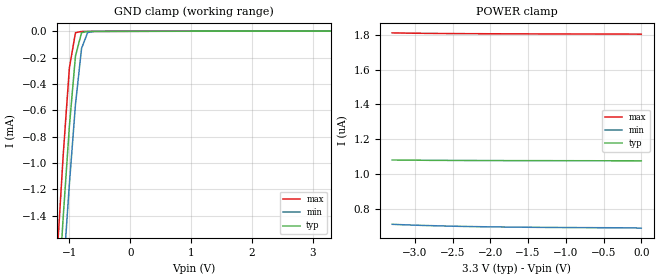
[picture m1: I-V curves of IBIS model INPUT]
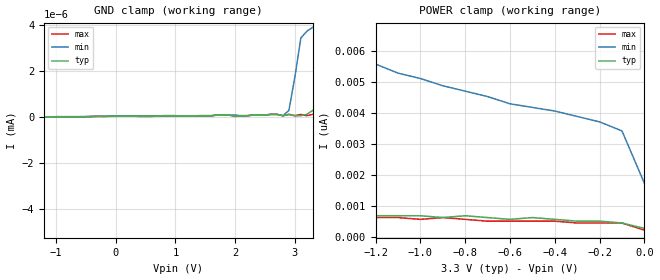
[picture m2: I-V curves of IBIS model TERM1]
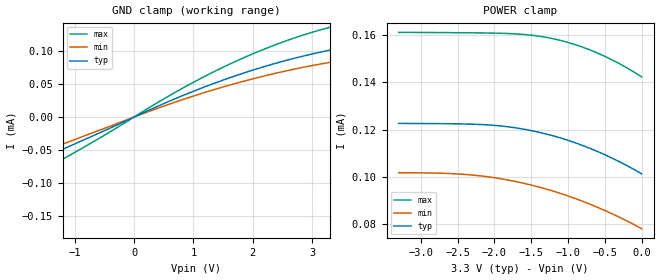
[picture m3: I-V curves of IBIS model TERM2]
|   PERICOM SEMICONDUCTOR CORP
|   IBIS Model of PI3USB223
|   Product Family: 3USB
|   UQFN (ZM) Package
[IBIS Ver] 3.2
[Comment char] |_char
[File Name] pi3usb223_zm_33v.ibs
[File Rev] 1.0
[Source] File originated at Pericom Semiconductor Corp.
[Date] 9/17/15
[Disclaimer] (C) Copyright PERICOM Semiconductor Corporation
   All rights reserved
  Pericom Semiconductor Corporation hereby grants the user of
  this IBIS model a non-exclusive, nontransferable license to
  use this IBIS model under the following terms.
  This IBIS model is provided on an "AS IS" basis and Pericom
  makes absolutely no warranty with respect to the information
  contained herein. PERICOM DISCLAIMS AND CUSTOMER WAIVES ALL
  WARRANTIES, EXPRESSED OR IMPLIED, INCLUDING WARRANTIES OF
  MERCHANTABILITY OR FITNESS FOR A PARTICULAR PURPOSE. The
  entire risk as to quality and performance is with the customer.
  Accordingly, in no event shall the company be liable for any
  damages, whether in contract or tort, including any lost
  profits or other incidental, consequential, exemplary, or
  punitive damages arising out of the use or application of the
  IBIS model provided in this package. Further, Pericom reserves
  the right to make changes without notice to any product herein
  to improve reliability, function, or design. Pericom does not
  convey any license under patent rights or any other intellectual
  property rights, including those of third parties.
  The user is granted this license only to use the IBIS model
  and is not granted rights to sell, load, rent, lease or license
  the IBIS model in whole or in part, or in modified form to anyone
  other than user. User may modify the IBIS model to suit its specific
  application but rights to derivative works and such modifications
  shall belong to Pericom.
  Pericom is not obligated to provide maintenance or support
  for the licensed IBIS model.
  Contact Pericom at ATTN: APPLICATION ENGINEERING / IBIS MODELS
  1545 Barber Lane Milpitas, CA 95035 USA.
[Component] PI3USB223
[Manufacturer] Pericom Semiconductor Corp.
[Package]
| variable   typ   min   max
R_pkg   0.028337ohm   0.027528ohm   0.029145ohm
L_pkg   0.39561nH   0.38133nH   0.40988nH
C_pkg   0.047513pF   0.038136pF   0.056889pF
[Pin]   signal_name   model_name   R_pin   L_pin   C_pin
1   D-   TERM1   0.027896   0.38515nH   0.041595pF
2   R   TERM2   0.027896   0.38515nH   0.041595pF
3   L   TERM2   0.029145   0.40988nH   0.056889pF
4   GND   GND   0.027528   0.38133nH   0.038136pF
5   VDD   POWER   0.029145   0.40988nH   0.056889pF
6   D-/L   TERM3   0.027896   0.38515nH   0.041595pF
7   D+/R   TERM3   0.027896   0.38515nH   0.041595pF
8   ASEL   INPUT   0.029145   0.40988nH   0.056889pF
9   VBUS   INPUT   0.027528   0.38133nH   0.038136pF
10   D+   TERM1   0.029145   0.40988nH   0.056889pF
[Series Switch Groups]
On 1 /
Off 2 /
[Series Pin Mapping]   pin_2   model_name  function_table_group
1   6   SWITCH1   1
10   7   SWITCH1   1
2   6   SWITCH2   2
3   7   SWITCH2   2
|   Model SWITCH1
[Model] SWITCH1
Model_type Series_switch
| variable   typ   min   max
C_comp   7.000pF   6.900pF   7.100pF
[Voltage Range]   3.300V   3.000V   3.600V
[GND Clamp Reference]   0.000V   0.000V   0.000V
[POWER Clamp Reference]   3.300V   3.000V   3.600V
[On]
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[OFF]
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|   Model SWITCH2
[Model] SWITCH2
Model_type Series_switch
| variable   typ   min   max
C_comp   7.000pF   6.900pF   7.100pF
[Voltage Range]   3.300V   3.000V   3.600V
[GND Clamp Reference]   0.000V   0.000V   0.000V
[POWER Clamp Reference]   3.300V   3.000V   3.600V
[On]
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[OFF]
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| Models and submodels in the file (6): INPUT (Input), SWITCH1 (Series_switch), SWITCH2 (Series_switch), TERM1 (Terminator), TERM2 (Terminator), TERM3 (Terminator)
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|   Model INPUT
[Model] INPUT
Model_type Input
Vinl = 0.800V
Vinh = 2.000V
| variable   typ   min   max
C_comp   1.000pF   0.900pF   1.100pF
[Voltage Range]   3.300V   3.000V   3.600V
[GND Clamp Reference]   0.000V   0.000V   0.000V
[POWER Clamp Reference]   3.300V   3.000V   3.600V
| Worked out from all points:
|   GND clamp passes 1 mA (typ) near -1.04 V on its own axis
[GND Clamp]
| Voltage   I(typ)   I(min)   I(max)
-3.3V     -19.61mA   -19.28mA   -20.05mA
-1.2V     -2.136mA   -2.542mA   -1.694mA
-1.1V     -1.403mA   -1.835mA   -931.7uA
-1V       -721.6uA   -1.161mA   -278uA
-900mV    -187.7uA   -555.9uA   -10.55uA
-800mV    -10.15uA   -129.5uA   -1.14uA
-700mV    -880.6nA   -9.377uA   -929.6nA
-500mV    -459.5nA   -365.8nA   -657.3nA
3.3V      1.076uA    692.4nA    1.803uA
[POWER Clamp]   |Note: Vtable = Vcc - Voutput
| Voltage   I(typ)   I(min)   I(max)
-3.3V     1.081uA    712.6nA    1.81uA
-3.2V     1.081uA    710.6nA    1.81uA
-3.1V     1.08uA     709.1nA    1.809uA
-3V       1.08uA     707.6nA    1.808uA
-2.8V     1.079uA    704.9nA    1.808uA
-2.5V     1.079uA    701.6nA    1.806uA
-2.1V     1.078uA    698.4nA    1.805uA
-1.5V     1.077uA    695.5nA    1.805uA
-1.3V     1.077uA    694.8nA    1.804uA
-1V       1.077uA    693.9nA    1.804uA
-100mV    1.077uA    691.9nA    1.803uA
0V        1.076uA    690.3nA    1.803uA
|   Model TERM1
[Model] TERM1
Model_type Terminator
| variable   typ   min   max
C_comp   3.000pF   2.950pF   3.050pF
[Voltage Range]   3.300V   3.000V   3.600V
[GND Clamp Reference]   0.000V   0.000V   0.000V
[POWER Clamp Reference]   3.300V   3.000V   3.600V
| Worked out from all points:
|   GND clamp passes 1 mA (typ) near -2.90 V on its own axis
[GND Clamp]
| Voltage   I(typ)   I(min)   I(max)
-3.3V     -1.584A    -1.988A    -1.092A
-2.5V     -307nA     -2.561uA   -8.702nA
-2.4V     -10.74nA   -165.2nA   -116.4pA
-2.3V     -349.2pA   -8.702nA   0A
-2.2V     -58.21pA   -407.5pA   0A
-2.1V     0A         -58.21pA   0A
2.6V      116.4pA    116.4pA    116.4pA
2.8V      58.21pA    58.21pA    58.21pA
2.9V      116.4pA    291pA      116.4pA
3V        58.21pA    1.746nA    58.21pA
3.1V      58.21pA    3.434nA    116.4pA
3.3V      291pA      3.9nA      116.4pA
[POWER Clamp]   |Note: Vtable = Vcc - Voutput
| Voltage   I(typ)   I(min)   I(max)
-3.3V     1.63nA     21.77nA    1.048nA
-3.1V     1.513nA    18.86nA    814.9pA
-2.9V     1.513nA    16.18nA    814.9pA
-2.8V     1.281nA    15.02nA    931.3pA
-2.6V     1.164nA    13.04nA    931.3pA
-2.5V     1.164nA    11.99nA    698.5pA
-2.2V     931.3pA    9.895nA    814.9pA
-2.1V     1.048nA    9.313nA    698.5pA
-1.5V     873.1pA    6.519nA    640.3pA
-1.1V     698.5pA    5.297nA    640.3pA
-100mV    465.7pA    3.434nA    465.7pA
0V        291pA      1.746nA    232.8pA
|   Model TERM2
[Model] TERM2
Model_type Terminator
| variable   typ   min   max
C_comp   3.000pF   2.950pF   3.050pF
[Voltage Range]   3.300V   3.000V   3.600V
[GND Clamp Reference]   0.000V   0.000V   0.000V
[POWER Clamp Reference]   3.300V   3.000V   3.600V
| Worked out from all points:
|   GND clamp passes 1 mA (typ) near -2.87 V on its own axis
[GND Clamp]
| Voltage   I(typ)   I(min)   I(max)
-3.3V     -1.929A    -2.461A    -1.311A
-2.8V     -415.1uA   -964.9uA   -291.1uA
-2.7V     -158uA     -227.9uA   -148.8uA
-2.6V     -107.8uA   -107.1uA   -132.8uA
-2.5V     -100.4uA   -88.46uA   -128uA
-2.4V     -96.58uA   -83.78uA   -123.6uA
-2.1V     -85.53uA   -73.62uA   -110uA
-800mV    -32.74uA   -27.27uA   -43.25uA
200mV     8.325uA    6.783uA    11.2uA
1.3V      49.35uA    40.18uA    66.52uA
2.3V      79.11uA    64.47uA    106.5uA
3.3V      101.2uA    82.7uA     135.8uA
[POWER Clamp]   |Note: Vtable = Vcc - Voutput
| Voltage   I(typ)   I(min)   I(max)
-3.3V     122.6uA    101.7uA    161.3uA
-2.6V     122.5uA    101.3uA    161.2uA
-2.2V     122.2uA    100.3uA    161.1uA
-1.9V     121.5uA    99.02uA    160.9uA
-1.7V     120.7uA    97.84uA    160.6uA
-1.5V     119.6uA    96.42uA    160.1uA
-1.3V     118.1uA    94.75uA    159.2uA
-1V       115.4uA    91.79uA    157uA
-800mV    113.2uA    89.5uA     155uA
-600mV    110.7uA    86.97uA    152.5uA
-300mV    106.3uA    82.7uA     148uA
0V        101.2uA    77.88uA    142.4uA
